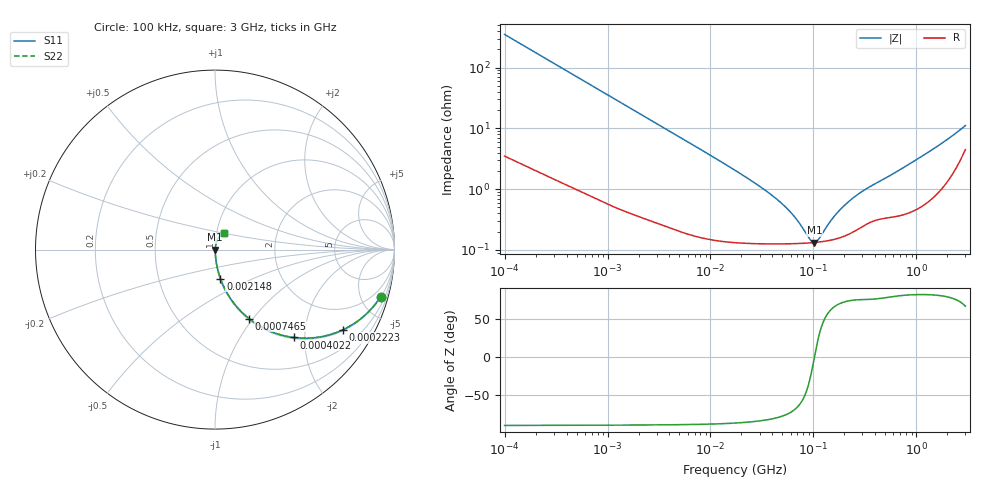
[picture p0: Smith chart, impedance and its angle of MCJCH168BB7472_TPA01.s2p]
! MCJCH168BB7472_TPA01  S-PARAMETER MODEL  ( Standard Model )
! Model Generated by TAIYO YUDEN Corporation (http://www.ty-top.com)
! Version 1.0
! TAIYO YUDEN Control No. 220601
! Copyright(c) 2015 TAIYO YUDEN CO.,LTD. All Rights Reserved.
! Product Description (link to TY-COMPAS)
! https://ds.yuden.co.jp/TYCOMPAS/or/detail?pn=MCJCH168BB7472KTPA01&u=M
! Products Name : Multilayer Ceramic Capacitors
! Characteristics :
!  Capacitance : 4700 [pF] , Rated Voltage : 100 [V] , TCC : X7R
!  Case Size : 1.6 x 0.8 / 0.063 x 0.031 [mm/inch] , Thickness : 0.8 / 0.031 [mm/inch]
!  (Conditions: Temperature = 25 [degC] , DC Bias Voltage = 0 [V])
! External Node Assignments :
!  1  o---| |---o  2
! GND o---------o GND
! Frequency Range : 100kHz  -  3GHz  [ 401 STEP ]
# MHZ S RI R 50
! Freq[MHz].  S11 Real  S11 Imag  S21 Real  S21 Imag  S12 Real  S12 Imag  S22 Real  S22 Imag
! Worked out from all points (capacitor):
!   401 points, 100 kHz to 3 GHz, reference 50 ohm
!   read as one part in series: C = 4.53 nF near 105.3 kHz
!   lowest |Z| = 133 mohm at 102.5 MHz (marker M1)
!   series resonance near 102.5 MHz, so ESL is about 530 pH
!   S11 on the Smith chart (normalised r, x): 100 kHz: 1.07, -7.01; 222.3 kHz: 1.04, -3.17; 402.2 kHz: 1.02, -1.76; 746.5 kHz: 1.01, -0.95; 2.148 MHz: 1.01, -0.33; 3 GHz: 1.09, +0.20
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0.1  0.9226 -0.2623  0.0774 0.2623  0.0774 0.2623  0.9226 -0.2623
0.151038  0.8415 -0.3598  0.1585 0.3598  0.1585 0.3598  0.8415 -0.3598
0.222319  0.7132 -0.4465  0.2868 0.4465  0.2868 0.4465  0.7132 -0.4465
0.402172  0.4375 -0.4895  0.5625 0.4895  0.5625 0.4895  0.4375 -0.4895
0.562235  0.2878 -0.4457  0.7122 0.4457  0.7122 0.4457  0.2878 -0.4457
0.746515  0.1888 -0.3839  0.8112 0.3839  0.8112 0.3839  0.1888 -0.3839
1.18716  0.0868 -0.2734  0.9132 0.2734  0.9132 0.2734  0.0868 -0.2734
2.147551  0.0303 -0.1615  0.9697 0.1615  0.9697 0.1615  0.0303 -0.1615
3.161081  0.0154 -0.1119  0.9846 0.1119  0.9846 0.1119  0.0154 -0.1119
17.7727  0.00171 -0.0198  0.9983 0.0198  0.9983 0.0198  0.00171 -0.0198
33.85116  0.00135 -0.00957  0.9986 0.00957  0.9986 0.00957  0.00135 -0.00957
51.12795  0.00129 -0.00535  0.9987 0.00535  0.9987 0.00535  0.00129 -0.00535
67.88584  0.00128 -0.00301  0.9987 0.00301  0.9987 0.00301  0.00128 -0.00301
97.38194  0.00132 -0.000365  0.9987 0.000365  0.9987 0.000365  0.00132 -0.000365
102.5331  0.00133 2.07e-06  0.9987 -2.07e-06  0.9987 -2.07e-06  0.00133 2.07e-06
113.6672  0.00135 0.000737  0.9987 -0.000737  0.9987 -0.000737  0.00135 0.000737
163.0551  0.00152 0.00342  0.9985 -0.00342  0.9985 -0.00342  0.00152 0.00342
216.4987  0.00182 0.0058  0.9982 -0.0058  0.9982 -0.0058  0.00182 0.0058
310.5665  0.00259 0.00924  0.9974 -0.00924  0.9974 -0.00924  0.00259 0.00924
547.5153  0.00365 0.016  0.9963 -0.016  0.9963 -0.016  0.00365 0.016
1791.7  0.0134 0.0554  0.9866 -0.0554  0.9866 -0.0554  0.0134 0.0554
3000  0.0519 0.0923  0.9481 -0.0923  0.9481 -0.0923  0.0519 0.0923
